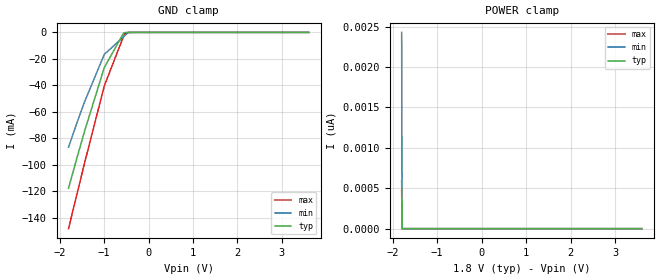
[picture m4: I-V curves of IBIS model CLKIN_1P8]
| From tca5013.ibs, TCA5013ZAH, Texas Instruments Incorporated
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|   Model CLKIN
[Model]   CLKIN_1P8
Model_type   Input
Vinl = .36
Vinh = 1.44
|   typ   min   max
C_comp   0.731p   0.503p   0.930p
[Model spec]
|subparameter
Vinl   0.36   0.33   0.39
Vinh   1.44   1.32   1.56
[Voltage Range]   1.8   1.65   1.95
[Temperature Range]   27   125   -40
[Power Clamp Reference]   1.8   1.65   1.95
[GND Clamp Reference]   0   0   0
[GND Clamp]
|   Voltage   I(typ)   I(min)   I(max)
-1.8V     -117.8mA   -86.81mA   -148.4mA
-1.438V   -74.52mA   -52.39mA   -98.64mA
-995.4mV  -26.56mA   -16.63mA   -40.42mA
-560.5mV  -436.9uA   -3.265mA   -2.757mA
-540mV    -282uA     -2.634mA   -981.4uA
-455.4mV  -35.54uA   -34.4uA    -116.2uA
3.6V      0A         0A         0A
[POWER Clamp]
|   Voltage   I(typ)   I(min)   I(max)
-1.8V     600.8pA    2.429nA    466.4pA
-1.789V   0A         0A         0A
-1.784V   0A         0A         0A
3.6V      0A         0A         0A
